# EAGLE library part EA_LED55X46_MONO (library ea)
ELECRONIC ASSEMBLY GmbH EA LED55x46-A EA LED55x46-B EA LED55x46-G EA LED55x46-R EA LED55x46-W
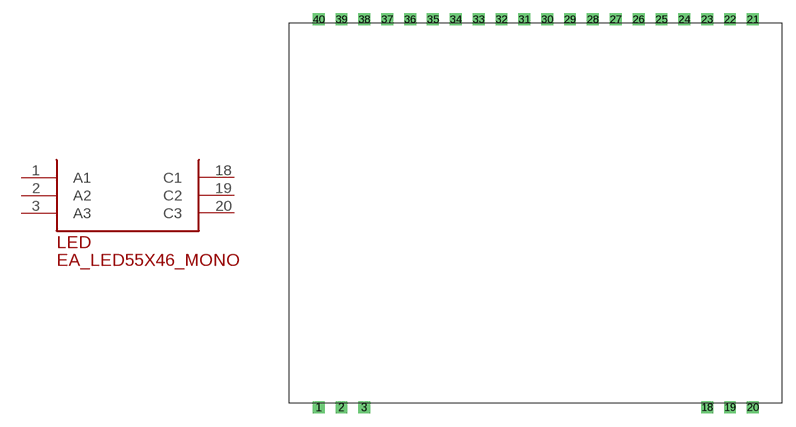
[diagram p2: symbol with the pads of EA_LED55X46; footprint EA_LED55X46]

Designator prefix LED

## EA_LED55X46_MONO  [EA_LED55X46]
1  A1  pas
2  A2  pas
3  A3  pas
18  C1  pas
19  C2  pas
20  C3  pas

## Footprint EA_LED55X46 (pad centres in mm)
drill 0.813 square: 1 0,0; 2 2.54,0; 3 5.08,0; 18 43.18,0; 19 45.72,0; 20 48.26,0; 21 48.26,43.18; 22 45.72,43.18; 23 43.18,43.18; 24 40.64,43.18; 25 38.1,43.18; 26 35.56,43.18; 27 33.02,43.18; 28 30.48,43.18; 29 27.94,43.18; 30 25.4,43.18; 31 22.86,43.18; 32 20.32,43.18; 33 17.78,43.18; 34 15.24,43.18; 35 12.7,43.18; 36 10.16,43.18; 37 7.62,43.18; 38 5.08,43.18; 39 2.54,43.18; 40 0,43.18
